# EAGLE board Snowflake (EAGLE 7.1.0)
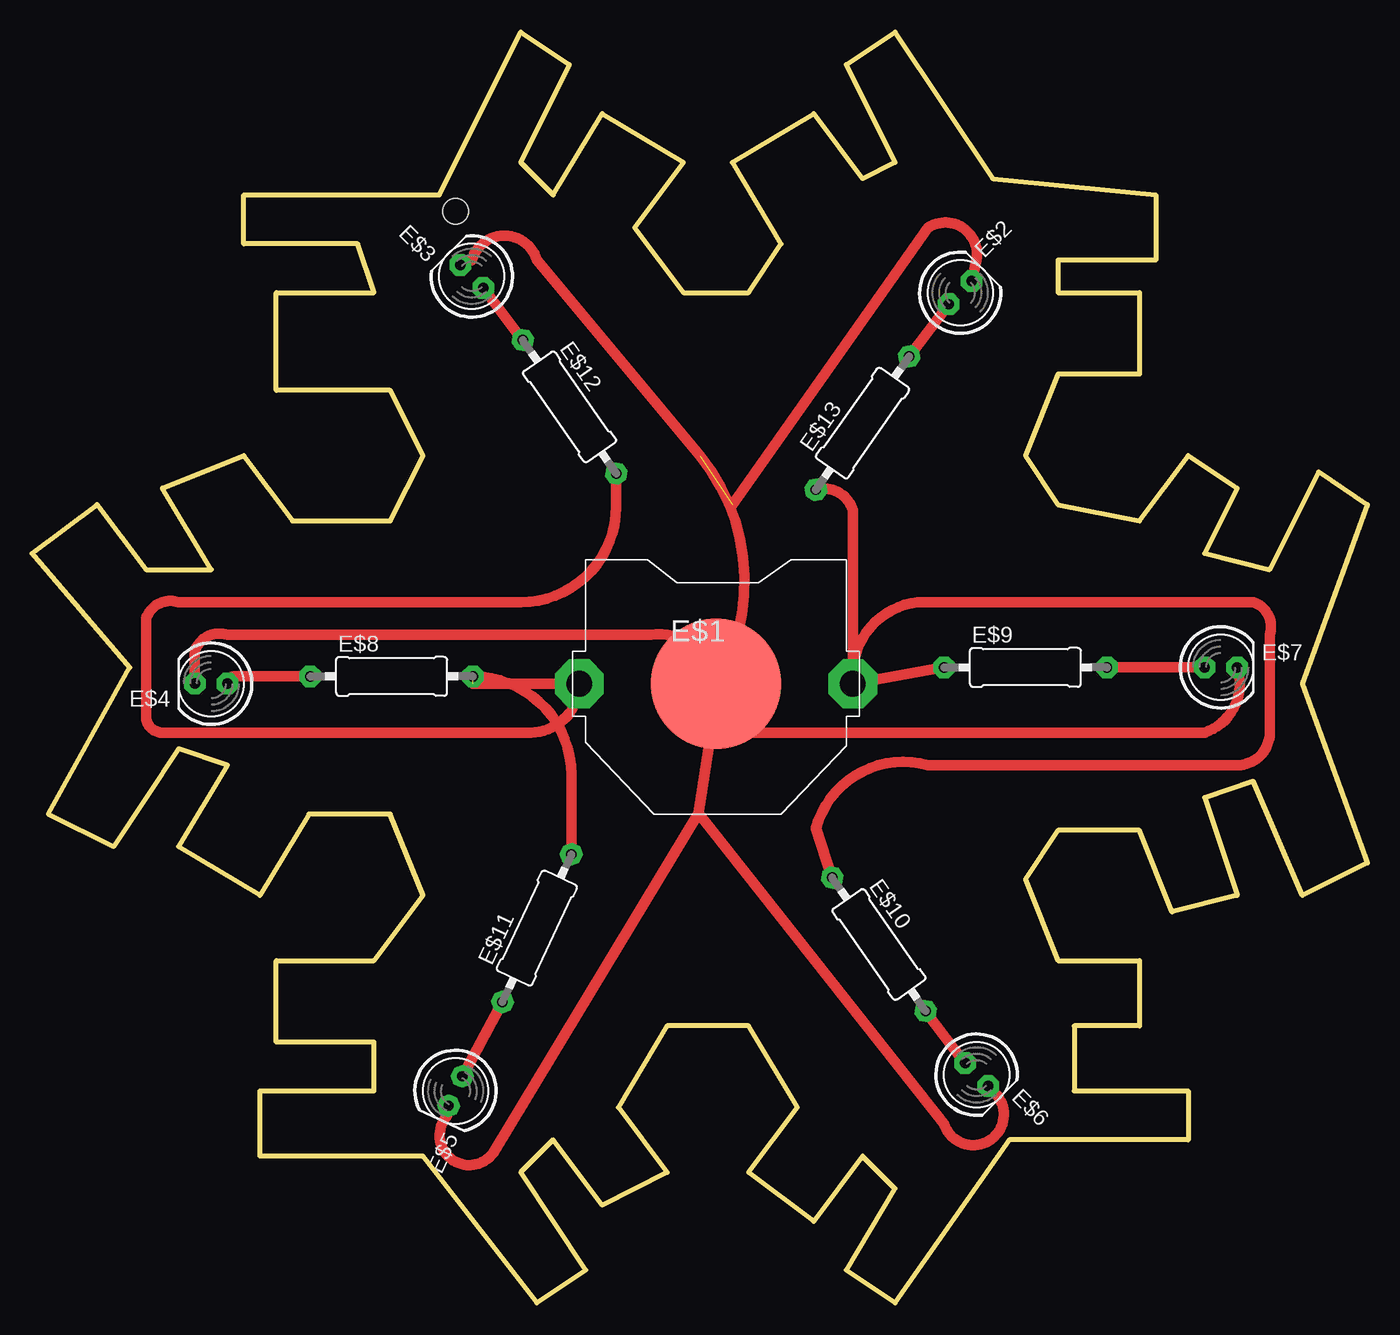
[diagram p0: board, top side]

Size 104.14 x 99.06 mm. Coordinates in mm from the lower left corner, seen from the top.
Outline: 102 segments
Copper layers (1*16): Top 0.035mm / dielectric 1.5mm / Bottom 0.035mm
Design rules "OthermillDRC_1_32_v2": minimum track width 8mil, minimum drill 0.8mm, track to track 0.794003125mm, track to pad 0.794003125mm, pad to pad 0.794003125mm, via to via 0.794003125mm, smd to smd 0mil, copper to edge 0mil, drill to drill 1mil, minimum pad ring 10mil, minimum via ring 10mil, stop-mask expansion 1mil, vias tented up to drill 30mil, thermal gap 10mil
Holes 2 mm at 33.02,85.09

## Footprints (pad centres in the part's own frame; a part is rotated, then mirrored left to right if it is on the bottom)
CR2032-THRU = drill 2 pad 3.81 octagon: +1 -10.668,0; +2 10.668,0 | smd 10.16 x 10.16: - 0,0
LED5MM = drill 0.813 pad 1.676 octagon: A -1.27,0; K 1.27,0
0309/12 = drill 0.813 pad 1.676 octagon: 1 -6.35,0; 2 6.35,0

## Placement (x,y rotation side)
E$1  [CR2032-THRU]  53.34,48.26 0 top
E$2  [LED5MM]  72.39,78.74 45 top
E$3  [LED5MM]  34.29,80.01 135 top
E$4  [LED5MM]  13.97,48.26 180 top
E$5  [LED5MM]  33.02,16.51 245 top
E$6  [LED5MM]  73.66,17.78 315 top
E$7  [LED5MM]  92.71,49.53 0 top
E$8  [0309/12]  28.04,48.83 0 top
E$9  [0309/12]  77.47,49.53 0 top
E$10  [0309/12]  66.04,27.94 305 top
E$11  [0309/12]  39.37,29.21 65 top
E$12  [0309/12]  41.91,69.85 305 top
E$13  [0309/12]  64.77,68.58 55 top

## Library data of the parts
E$1-E$13 = adafruit

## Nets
S$1: E$1.+1 E$8.2 E$11.2 E$12.2
S$2: E$4.A E$8.1
S$3: E$1.- E$2.K E$3.K E$4.K E$5.K E$6.K E$7.K
S$4: E$1.+2 E$9.1 E$10.1 E$13.1
S$5: E$7.A E$9.2
S$6: E$5.A E$11.1
S$7: E$3.A E$12.1
S$8: E$2.A E$13.2
S$9: E$6.A E$10.2

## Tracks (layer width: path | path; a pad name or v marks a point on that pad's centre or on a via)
S$1  (1 unrouted)
  Top 0.813: 34.39,48.26 E$1.+1 arc-90 38.86,44.45 10.16,44.45 arc-90 8.89,45.72 8.89,53.34 arc-90 11.43,54.61 38.1,54.61 arc90 45.55,62.06 E$12.2 | E$8.2 arc-90 42.05,41.17 E$11.2
S$2
  Top 0.813: E$4.A arc-90 15.81,48.83 E$8.1
S$3  (1 unrouted)
  Top 0.813: E$1.- arc90 48.26,52.07 15.24,52.07 arc90 12.7,50.8 E$4.K | E$7.K arc-90 91.44,44.45 53.34,44.45 53.34,46.99 | 53.34,46.99 E$1.- | E$5.K 32.38,14.61 arc197 36.2,12.07 51.97,38.15 | 51.97,38.15 53.34,46.99 | E$3.K 34.29,81.28 arc-148 39.37,81.28 52.07,66.04 arc-70 E$1.- | E$2.K 73.66,81.28 arc133 69.85,83.82 54.61,62.23 | E$6.K 74.93,16.51 arc-213 71.12,13.97 51.97,38.15
S$4
  Top 0.813: E$1.+2 E$9.1 | E$1.+2 64.01,61.77 arc90 E$13.1 | E$1.+2 arc-90 69.09,54.61 95.25,54.61 arc-90 96.52,52.07 96.52,44.45 arc-90 93.98,41.91 69.85,41.91 arc90 61.13,37 E$10.1
S$5
  Top 0.813: E$9.2 E$7.A
S$6
  Top 0.813: E$11.1 E$5.A
S$7
  Top 0.813: E$12.1 E$3.A
S$8
  Top 0.813: E$13.2 E$2.A
S$9
  Top 0.813: E$10.2 E$6.A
